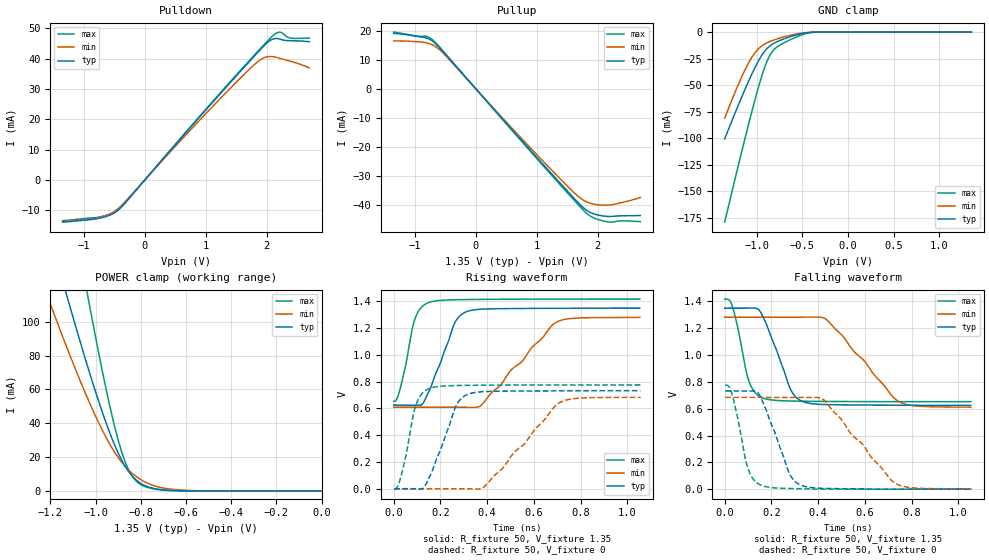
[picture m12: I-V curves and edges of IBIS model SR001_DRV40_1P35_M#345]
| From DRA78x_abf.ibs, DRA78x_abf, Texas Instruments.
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| Model based on original model for DDR_DIFFIOPB_V
|   Sub model SR001_DRV40_1P35
[model]   SR001_DRV40_1P35_M#345
|[Description]  [1.35V-I/O-X-X]
|   , ,
|[Input Load]
|[Output Drive]
|Voltage   1.35V
|Mode   I/O
Model_type   I/O
Polarity   Non-Inverting
Enable   Active-Low
Vinl =  0.585
Vinh =  0.765
Cref =  15.0000pF
Rref =  100.0000M
Vref =  0V
Vmeas =  0.675
C_comp   2p   2p   2p
[Model Spec]
Vinl   0.585   0.55125   0.61875
Vinh   0.765   0.73125   0.79875
[Receiver Thresholds]
Tslew_ac = 5n
Vth = 0.675
Vth_max = 0.709
Vth_min = 0.608
Vinh_ac = 0.175
Vinh_dc = 0.1
Vinl_ac = -0.175
Vinl_dc = -0.1
[Temperature Range]   25   125   -40
[Voltage Range]   1.35   1.2825   1.4175
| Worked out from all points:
|   slope of the pulldown table from 0 to 0.203 V, typ, clamps not added: 43 ohm
|   slope of the pullup table from 0 to 0.203 V, typ, clamps not added: 42 ohm
|   GND clamp passes 1 mA (typ) near -0.48 V on its own axis
|   POWER clamp passes 1 mA (typ) near -0.72 V on its own axis
|   rising waveform, R_fixture 50, V_fixture 1.35: 20-80 % time 91.2ps typ, 208ps min, 54.4ps max; typ from 0.625 V to 1.35 V
|   rising waveform, R_fixture 50, V_fixture 0: 20-80 % time 91.2ps typ, 202ps min, 54.1ps max; typ from 0 V to 0.733 V
|   falling waveform, R_fixture 50, V_fixture 1.35: 20-80 % time 91.3ps typ, 193ps min, 55.5ps max; typ from 1.35 V to 0.625 V
|   falling waveform, R_fixture 50, V_fixture 0: 20-80 % time 91.2ps typ, 197ps min, 55.2ps max; typ from 0.733 V to 0 V
[POWER_clamp]
-1.35V    224.4mA    165.8mA    358.5mA
-1.214V   157mA      115.5mA    250.8mA
-1.132V   117.8mA    86.59mA    187.7mA
-1.118V   111.4mA    81.92mA    177.3mA
-1.036V   74.26mA    55.16mA    116.8mA
-954.5mV  40.7mA     31.91mA    61.06mA
-900mV    22.42mA    19.79mA    30.14mA
-859.1mV  12.48mA    13.09mA    13.96mA
-804.5mV  4.85mA     7.084mA    4.132mA
-736.4mV  1.313mA    2.9mA      1.073mA
-627.3mV  101.6uA    577.3uA    45.9uA
0V        75.63nA    322.4nA    418.5nA
[Pulldown]
-1.35V    -13.93mA   -13.71mA   -13.45mA
-736.4mV  -12.58mA   -12.32mA   -12.19mA
-531.8mV  -11.22mA   -10.8mA    -10.99mA
-409.1mV  -9.378mA   -8.926mA   -9.416mA
1.145V    26.32mA    24.88mA    26.57mA
1.718V    39.05mA    36.49mA    39.37mA
1.923V    43.49mA    39.91mA    43.83mA
2.005V    45.12mA    40.54mA    45.58mA
2.086V    46.28mA    40.65mA    47.24mA
2.209V    46.44mA    40.1mA     48.7mA
2.373V    45.86mA    39.19mA    46.8mA
2.7V      45.54mA    36.91mA    46.74mA
[Pullup]
-1.35V    19.14mA    16.53mA    19.57mA
-981.8mV  18.13mA    16.28mA    18.23mA
-818.2mV  17.57mA    15.91mA    18.13mA
-736.4mV  16.82mA    15.4mA     17.33mA
-613.6mV  14.56mA    13.83mA    14.83mA
1.064V    -25.08mA   -24.06mA   -25.52mA
1.555V    -36.41mA   -34.6mA    -37.03mA
1.759V    -40.9mA    -38.29mA   -41.73mA
1.923V    -42.98mA   -39.67mA   -44.36mA
2.127V    -43.9mA    -40.1mA    -45.7mA
2.291V    -43.85mA   -39.69mA   -45.73mA
2.7V      -43.64mA   -37.43mA   -45.74mA
[GND_clamp]
-1.35V    -100.7mA   -81.27mA   -179.3mA
-1.241V   -77.31mA   -57.61mA   -140mA
-1.132V   -54.83mA   -36.31mA   -101.6mA
-1.05V    -39.08mA   -23.36mA   -74mA
-968.2mV  -25.28mA   -14.71mA   -48.34mA
-913.6mV  -18.13mA   -11.32mA   -33.52mA
-859.1mV  -13.28mA   -9.024mA   -22.35mA
-831.8mV  -11.61mA   -8.091mA   -18.64mA
-777.3mV  -9.078mA   -6.444mA   -14.07mA
-531.8mV  -1.871mA   -1.307mA   -3.441mA
-368.2mV  -88.76uA   -111.2uA   -158uA
1.35V     75.63nA    385.5nA    349.4nA
[Ramp]
dV/dt_f 0.43558262/91.40583p  0.40476929/0.19325305n 0.45930907/55.547329p
dV/dt_r 0.44168804/91.627517p 0.41292997/0.20360653n 0.46732083/54.369436p
R_load = 50
[Rising Waveform]
R_fixture = 50
V_fixture = 1.35
V_fixture_min = 1.2825
V_fixture_max = 1.4175
0s        624.9mV    609.4mV    653.1mV
27.79ps   624.2mV    609.3mV    746.8mV
91.18ps   623.5mV    609.3mV    1.27V
121.3ps   629.9mV    609.3mV    1.361V
145.1ps   706.4mV    609.3mV    1.388V
259.6ps   1.233V     609.2mV    1.412V
310.9ps   1.323V     608.3mV    1.414V
375.5ps   1.342V     625.6mV    1.415V
698.2ps   1.349V     1.246V     1.417V
1.053ns   1.35V      1.282V     1.417V
[Rising Waveform]
R_fixture = 50
V_fixture = 0
V_fixture_min = 0
V_fixture_max = 0
2.607ps   0V         0V         0V
31.2ps    0V         0V         91.09mV
95.89ps   0V         0V         628mV
124ps     0V         0V         716.1mV
150.3ps   76.77mV    0V         747.6mV
264.9ps   611.5mV    0V         771.2mV
314ps     703.5mV    0V         772.7mV
389.8ps   726.1mV    18.78mV    773.9mV
711.8ps   731.9mV    644.7mV    775.5mV
1.055ns   733mV      684.9mV    775.7mV
[Falling Waveform]
R_fixture = 50
V_fixture = 1.35
V_fixture_min = 1.2825
V_fixture_max = 1.4175
0s        1.35V      1.282V     1.417V
20.88ps   1.35V      1.283V     1.408V
35.66ps   1.35V      1.283V     1.348V
105.4ps   1.35V      1.283V     797mV
160.7ps   1.296V     1.283V     681.5mV
279.8ps   751.5mV    1.283V     657.7mV
330.8ps   656mV      1.282V     656.1mV
437.1ps   630.7mV    1.262V     654.2mV
748.3ps   626.2mV    650.7mV    652.7mV
1.053ns   624.9mV    609.4mV    652.5mV
[Falling Waveform]
R_fixture = 50
V_fixture = 0
V_fixture_min = 0
V_fixture_max = 0
2.607ps   733mV      684.9mV    775.7mV
33.13ps   733.2mV    685mV      698.6mV
101ps     732.8mV    685mV      146.5mV
136.9ps   727.2mV    685mV      48.51mV
156.9ps   673.5mV    685mV      28.46mV
275.3ps   122.3mV    685mV      4.697mV
325.9ps   29.81mV    684.8mV    2.976mV
425.7ps   5.882mV    663.1mV    0V
732.2ps   0V         40.9mV     0V
1.055ns   0V         0V         0V
